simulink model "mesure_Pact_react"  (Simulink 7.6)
settings: Solver=ode23tb  StartTime=0.0  StopTime=0.2  RelTol=1e-3
InitFcn:
  | clc
  | clear all
  | close all
  | delete *.mat
StopFcn:
  | load Pact_React.mat
  | subplot 211
  | plot(x(1,:),x(2,:),x(1,:),x(3,:))
  | grid
  | %axis([0 0.04 -0.2 1.2])
  | title('commande gâchette')
  | xlabel('temps')
  | 
  | subplot 212
  | plot(x(1,:),x(4,:),x(1,:),x(5,:))
  | title('tension aux bornes de la charge R et sinusoïde d''entrée')
  | grid
  | xlabel('temps')
  | 
  | delete *.mat
libraries: powerlib x13, powerlib_extras x7

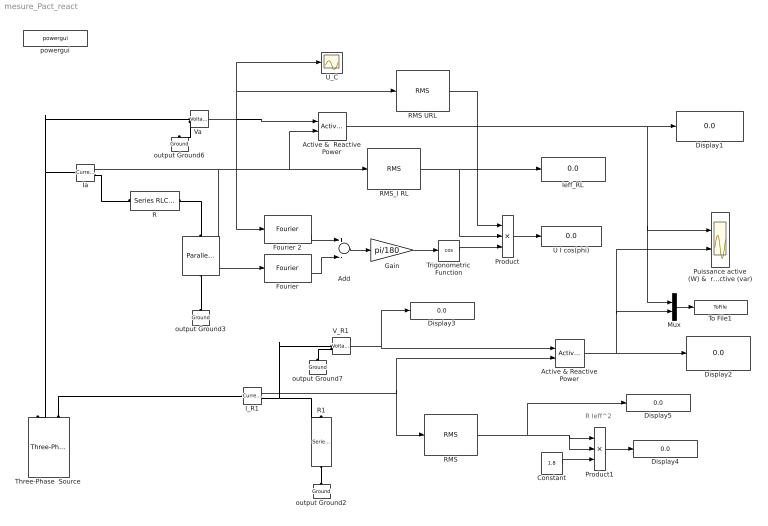
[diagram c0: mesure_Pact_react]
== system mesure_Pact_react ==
  note: R Ieff^2
  Active &  Reactive Power : powerlib_extras/Measurements/Active & Reactive Power  DialogController=POWERSYS.PowerSysDialog  SystemSampleTime=-1  f1=60
  Active & Reactive Power : powerlib_extras/Measurements/Active & Reactive Power  DialogController=POWERSYS.PowerSysDialog  SystemSampleTime=-1  f1=60
  Add : Sum  Inputs=+-
  Constant : Constant  Value=1.8
  Display{1..5} (5 alike) : Display
  Fourier : powerlib_extras/Measurements/Fourier  DialogController=POWERSYS.PowerSysDialog  SystemSampleTime=-1  f1=60  n=1
  Fourier 2 : powerlib_extras/Measurements/Fourier  DialogController=POWERSYS.PowerSysDialog  SystemSampleTime=-1  f1=60  n=1
  Gain : Gain  Gain=pi/180
  I_R1 : powerlib/Measurements/Current Measurement  Tag=PoWeRsYsTeMmEaSuReMeNt  DialogController=POWERSYS.PowerSysDialog  SystemSampleTime=-1  PhasorSimulation=off  OutputType=Magnitude  PSBequivalent=0
  Ia : powerlib/Measurements/Current Measurement  Tag=PoWeRsYsTeMmEaSuReMeNt  DialogController=POWERSYS.PowerSysDialog  SystemSampleTime=-1  PhasorSimulation=off  OutputType=Magnitude  PSBequivalent=0
  Ieff_RL : Display
  L : powerlib/Elements/Parallel RLC Branch  DialogController=POWERSYS.PowerSysDialog  PhysicalDomain=powersysdomain  SubClassName=unknown  LeftPortType=p1  RightPortType=p1  LConnTagsString=a  RConnTagsString=__new0  BranchType=L  Resistance=1  Inductance=1e-3  SetiL0=off  InitialCurrent=0  Capacitance=1e-6  Setx0=off  InitialVoltage=0  Measurements=None
  Mux : Mux  Inputs=2
  Product : Product  Inputs=3
  Product1 : Product  Inputs=3
  Puissance active (W) &  réactive (var) : Scope  NumInputPorts=2
  R : powerlib/Elements/Series RLC Branch  DialogController=POWERSYS.PowerSysDialog  PhysicalDomain=powersysdomain  SubClassName=unknown  LeftPortType=p1  RightPortType=p1  LConnTagsString=__new0  RConnTagsString=__new0  BranchType=R  Resistance=1  Inductance=1e-3  SetiL0=off  InitialCurrent=0  Capacitance=1e-6  Setx0=off  InitialVoltage=0  Measurements=None
  R1 : powerlib/Elements/Series RLC Branch  DialogController=POWERSYS.PowerSysDialog  PhysicalDomain=powersysdomain  SubClassName=unknown  LeftPortType=p1  RightPortType=p1  LConnTagsString=__new0  RConnTagsString=__new0  BranchType=R  Resistance=1.8  Inductance=1e-3  SetiL0=off  InitialCurrent=0  Capacitance=1e-6  Setx0=off  InitialVoltage=0  Measurements=None
  RMS : powerlib_extras/Measurements/RMS  DialogController=POWERSYS.PowerSysDialog  SystemSampleTime=-1  f1=60
  RMS URL : powerlib_extras/Measurements/RMS  DialogController=POWERSYS.PowerSysDialog  SystemSampleTime=-1  f1=60
  RMS_I RL : powerlib_extras/Measurements/RMS  DialogController=POWERSYS.PowerSysDialog  SystemSampleTime=-1  f1=60
  Three-Phase  Source : powerlib/Electrical Sources/Three-Phase Source  DialogController=POWERSYS.PowerSysDialog  SystemSampleTime=-1  Voltage=220  PhaseAngle=0  Frequency=60  InternalConnection=Yg  SpecifyImpedance=off  Resistance=0  Inductance=0  ShortCircuitLevel=100e6  BaseVoltage=25e3  XRratio=7
  To File1 : ToFile  Filename=Pact_React  MatrixName=x
  Trigonometric Function : Trigonometry  Operator=cos
  U I cos(phi) : Display
  U_C : Scope
  V_R1 : powerlib/Measurements/Voltage Measurement  Tag=PoWeRsYsTeMmEaSuReMeNt  DialogController=POWERSYS.PowerSysDialog  SystemSampleTime=-1  PhasorSimulation=off  OutputType=Magnitude  PSBequivalent=0
  "Va " : powerlib/Measurements/Voltage Measurement  Tag=PoWeRsYsTeMmEaSuReMeNt  DialogController=POWERSYS.PowerSysDialog  SystemSampleTime=-1  PhasorSimulation=off  OutputType=Magnitude  PSBequivalent=0
  output Ground{2..3,6..7} (4 alike) : powerlib/Elements/Ground  DialogController=POWERSYS.PowerSysDialog  PhysicalDomain=powersysdomain  SubClassName=unknown  LeftPortType=p1  RightPortType=p1  LConnTagsString=a
  powergui : powerlib/powergui  Priority=2  SystemSampleTime=-1  SimulationMode=Continuous  SampleTime=0  frequency=60  SPID=off  DisableSnubberDevices=off  DisableRonSwitches=off  DisableVfSwitches=off  SwTol=0  Interpol=off  frequencyindice=60  echomessages=off  HookPort=off  DisplayEquations=off  FunctionMessages=off  EnableUseOfTLC=off  x0status=blocks  RestoreLinks=warning  ResistiveCurrentMeasurement=off  Frange=logspace(0,3,50)  Ylog=off  Xlog=off  ShowGrid=off  save=off  variable=ZData  ZoomFFT=on  StartTime=0.0  cycles=1  DisplayStyle=off  fundamental=60  FreqAxis=off  MaxFrequency=1000  frequencyindicesteady=1  RmsSteady=1  display=off  Ts=0  methode=off
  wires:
  V_R1/1 -> Display3/1, Active & Reactive Power/1
  I_R1/1 -> Active & Reactive Power/2, RMS/1
  Active & Reactive Power/1 -> Display2/1, Puissance active (W) &  réactive (var)/2, Mux/2
  Active &  Reactive Power/1 -> Display1/1, Puissance active (W) &  réactive (var)/1, Mux/1
  RMS_I RL/1 -> Ieff_RL/1, Product/2
  Product/1 -> U I cos(phi)/1
  Gain/1 -> Trigonometric Function/1
  Trigonometric Function/1 -> Product/3
  RMS URL/1 -> Product/1
  Ia/1 -> RMS_I RL/1, Active &  Reactive Power/2, Fourier/1
  Fourier 2/2 -> Add/1
  Fourier/2 -> Add/2
  Add/1 -> Gain/1
  "Va "/1 -> Active &  Reactive Power/1, U_C/1, RMS URL/1, Fourier 2/1
  Constant/1 -> Product1/3
  Product1/1 -> Display4/1
  RMS/1 -> Product1/1, Product1/2, Display5/1
  Mux/1 -> To File1/1
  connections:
  "Va "/LConn2 -- output Ground6/LConn1
  output Ground7/LConn1 -- V_R1/LConn2
  Ia/LConn1 -- Three-Phase  Source/RConn1 -- "Va "/LConn1
  output Ground3/LConn1 -- L/RConn1
  Three-Phase  Source/RConn3 -- I_R1/LConn1
  I_R1/RConn1 -- R1/LConn1 -- V_R1/LConn1
  R1/RConn1 -- output Ground2/LConn1
  L/LConn1 -- R/LConn1
  Ia/RConn1 -- R/RConn1
